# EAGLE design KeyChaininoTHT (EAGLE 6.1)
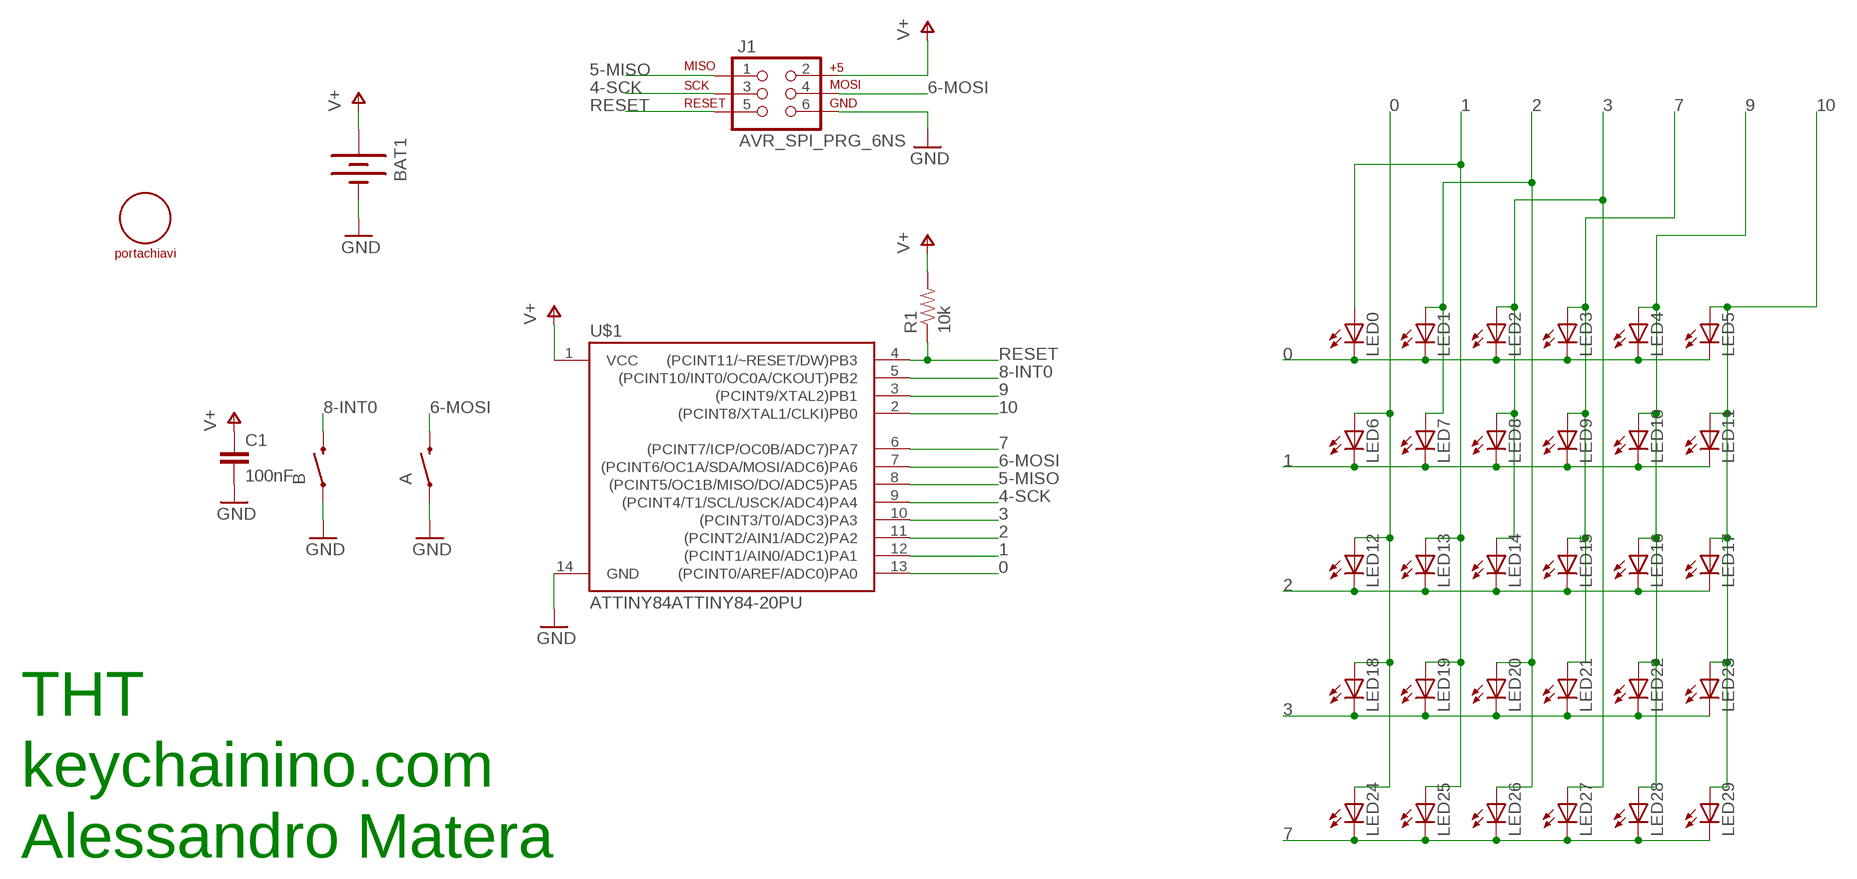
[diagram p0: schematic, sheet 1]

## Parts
A  SWITCH-MOMENTARY-2PTH  [TACTILE-PTH]
B  SWITCH-MOMENTARY-2PTH  [TACTILE-PTH]
BAT1  BATTERY20PTH  [BATTCOM_20MM_PTH]
C1  100nF  CAPPTH1  [CAP-PTH-5MM]
J1  AVR_SPI_PRG_6NS  [2X3-NS]
LED0  LED5MM-KIT  [LED5MM-KIT]
LED1  LED5MM-KIT  [LED5MM-KIT]
LED2  LED5MM-KIT  [LED5MM-KIT]
LED3  LED5MM-KIT  [LED5MM-KIT]
LED4  LED5MM-KIT  [LED5MM-KIT]
LED5  LED5MM-KIT  [LED5MM-KIT]
LED6  LED5MM-KIT  [LED5MM-KIT]
LED7  LED5MM-KIT  [LED5MM-KIT]
LED8  LED5MM-KIT  [LED5MM-KIT]
LED9  LED5MM-KIT  [LED5MM-KIT]
LED10  LED5MM-KIT  [LED5MM-KIT]
LED11  LED5MM-KIT  [LED5MM-KIT]
LED12  LED5MM-KIT  [LED5MM-KIT]
LED13  LED5MM-KIT  [LED5MM-KIT]
LED14  LED5MM-KIT  [LED5MM-KIT]
LED15  LED5MM-KIT  [LED5MM-KIT]
LED16  LED5MM-KIT  [LED5MM-KIT]
LED17  LED5MM-KIT  [LED5MM-KIT]
LED18  LED5MM-KIT  [LED5MM-KIT]
LED19  LED5MM-KIT  [LED5MM-KIT]
LED20  LED5MM-KIT  [LED5MM-KIT]
LED21  LED5MM-KIT  [LED5MM-KIT]
LED22  LED5MM-KIT  [LED5MM-KIT]
LED23  LED5MM-KIT  [LED5MM-KIT]
LED24  LED5MM-KIT  [LED5MM-KIT]
LED25  LED5MM-KIT  [LED5MM-KIT]
LED26  LED5MM-KIT  [LED5MM-KIT]
LED27  LED5MM-KIT  [LED5MM-KIT]
LED28  LED5MM-KIT  [LED5MM-KIT]
LED29  LED5MM-KIT  [LED5MM-KIT]
R1  10k  RESISTORPTH-1/4W  [AXIAL-0.4]
U$1  ATTINY84ATTINY84-20PU  [DIL14]
U$2  ANELLO-PORTACHIAVI  [HOLE-PORTACHIAVI]

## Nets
0: LED0.K(C) LED1.K(C) LED2.K(C) LED3.K(C) LED4.K(C) LED5.K(C) LED6.A LED12.A LED18.A LED24.A U$1.13((PCINT0/AREF/ADC0)PA0)
1: LED0.A LED6.K(C) LED7.K(C) LED8.K(C) LED9.K(C) LED10.K(C) LED11.K(C) LED13.A LED19.A LED25.A U$1.12((PCINT1/AIN0/ADC1)PA1)
2: LED1.A LED7.A LED12.K(C) LED13.K(C) LED14.K(C) LED15.K(C) LED16.K(C) LED17.K(C) LED20.A LED26.A U$1.11((PCINT2/AIN1/ADC2)PA2)
3: LED2.A LED8.A LED14.A LED18.K(C) LED19.K(C) LED20.K(C) LED21.K(C) LED22.K(C) LED23.K(C) LED27.A U$1.10((PCINT3/T0/ADC3)PA3)
4-SCK: J1.3 U$1.9((PCINT4/T1/SCL/USCK/ADC4)PA4)
5-MISO: J1.1 U$1.8((PCINT5/OC1B/MISO/DO/ADC5)PA5)
6-MOSI: A.3 J1.4 U$1.7((PCINT6/OC1A/SDA/MOSI/ADC6)PA6)
7: LED3.A LED9.A LED15.A LED21.A LED24.K(C) LED25.K(C) LED26.K(C) LED27.K(C) LED28.K(C) LED29.K(C) U$1.6((PCINT7/ICP/OC0B/ADC7)PA7)
8-INT0: B.3 U$1.5((PCINT10/INT0/OC0A/CKOUT)PB2)
9: LED4.A LED10.A LED16.A LED22.A LED28.A U$1.3((PCINT9/XTAL2)PB1)
10: LED5.A LED11.A LED17.A LED23.A LED29.A U$1.2((PCINT8/XTAL1/CLKI)PB0)
GND: A.1 B.1 BAT1.2(-) C1.2 J1.6 U$1.14(GND)
RESET: J1.5 R1.P$1 U$1.4((PCINT11/~RESET/DW)PB3)
V+: BAT1.1(+) C1.1 J1.2 R1.P$2 U$1.1(VCC)

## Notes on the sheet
- THT
- keychainino.com
- Alessandro Matera

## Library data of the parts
A B = SparkFun-Electromechanical:SWITCH-MOMENTARY-2: Various NO switches- pushbuttons, reed, etc
BAT1 = SparkFun-Electromechanical:BATTERY: Battery Holders
C1 = SparkFun-Passives:CAP: Capacitor
J1 = SparkFun-Connectors:AVR_SPI_PRG_6: AVR ISP 6 Pin This is the reduced ISP connector for AVR programming. Common on Arduino. This footprint will take up less PCB space and can be used with a 10-pin to 6-pin adapter such as SKU: BOB-08508
LED0 LED1-LED29 = SparkFun-LED:LED: LEDs
R1 = SparkFun-Resistors:RESISTOR: Resistor
U$1 = SparkFun-DigitalIC:ATTINY84: Atmel 14-pin 2/4/8kB flash uC
U$2 = anello-portachiavi:ANELLO-PORTACHIAVI

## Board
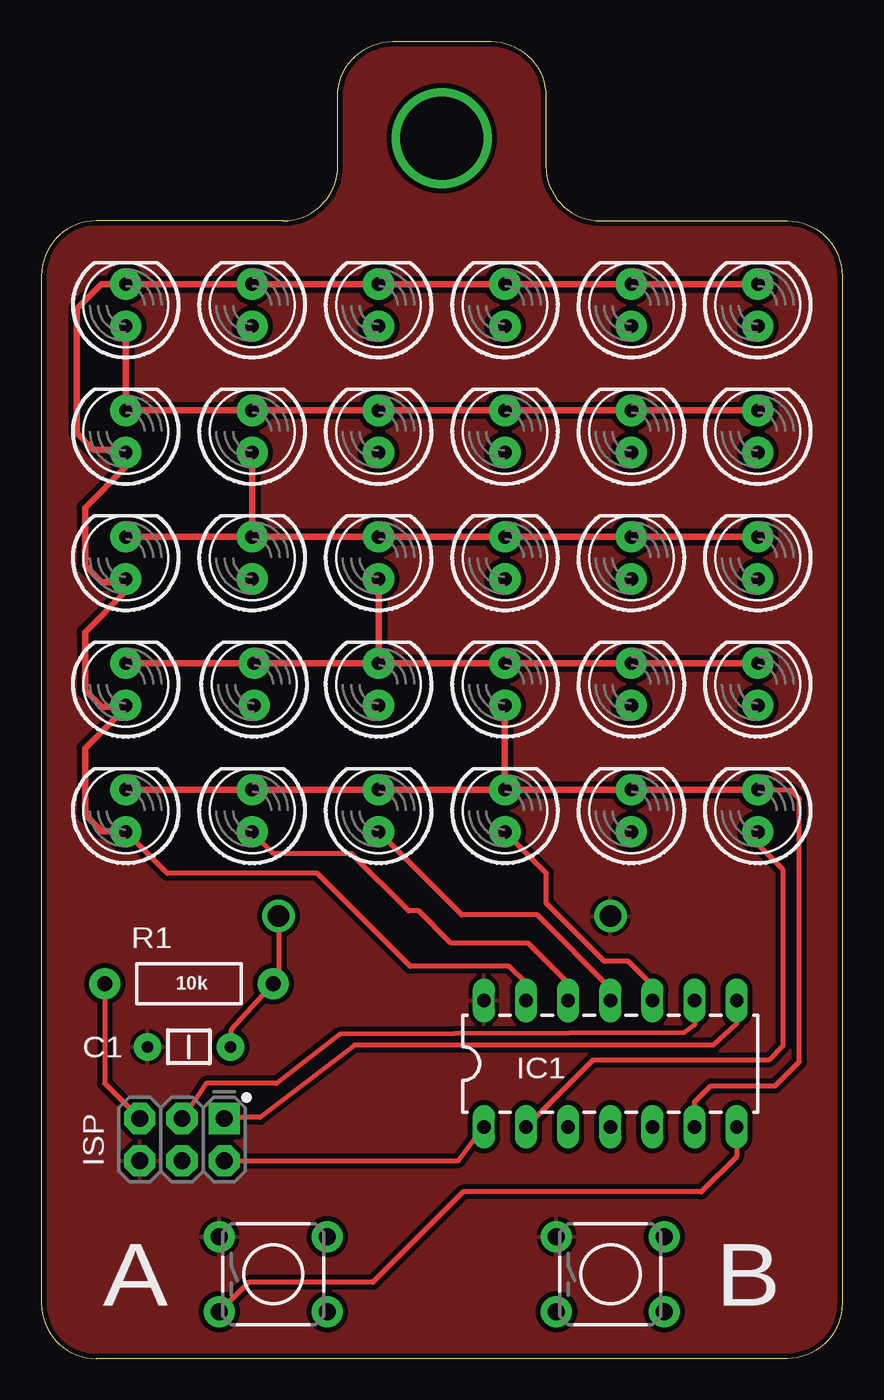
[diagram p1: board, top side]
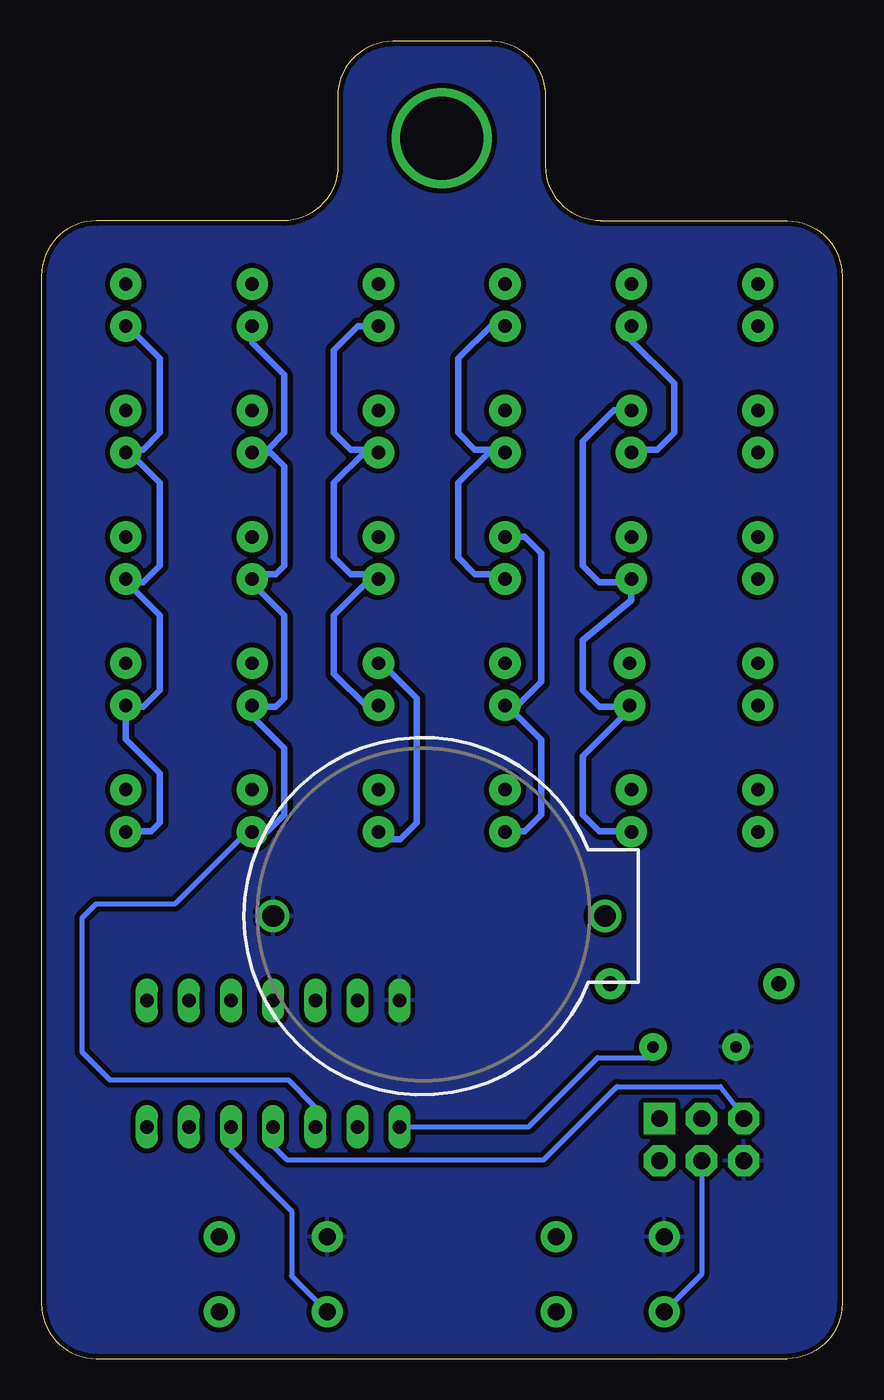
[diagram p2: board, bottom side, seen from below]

Size 48.26 x 79.39 mm. Coordinates in mm from the lower left corner, seen from the top.
Outline: 0,65.28 0,3.3 arc90 3.3,0 44.96,0 arc90 48.26,3.3 48.26,65.28 arc90 44.96,68.58 33.7,68.58 arc-90 30.4,71.88 30.4,76.09 arc90 27.1,79.39 21.16,79.39 arc90 17.86,76.09 17.86,71.88 arc-90 14.56,68.58 3.3,68.58 arc90 0,65.28
Copper layers (1*16): Top 0.035mm / dielectric 1.5mm / Bottom 0.035mm
Design rules: minimum track width 6mil, minimum drill 12mil, track to track 6mil, track to pad 6mil, pad to pad 6mil, via to via 6mil, smd to smd 0mil, copper to edge 10mil, drill to drill 10mil, minimum pad ring 10mil, minimum via ring 6mil, stop-mask expansion 2mil, vias tented up to drill 100mil, thermal gap 10mil

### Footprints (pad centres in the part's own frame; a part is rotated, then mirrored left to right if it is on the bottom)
TACTILE-PTH = drill 1.016 pad 1.88: 1 -3.251,2.261; 2 3.251,2.261; 3 -3.251,-2.261; 4 3.251,-2.261
BATTCOM_20MM_PTH = drill 1.3: 1 20,0; 2 0,0
CAP-PTH-5MM = drill 0.7 pad 1.651: 1 -2.5,0; 2 2.5,0
2X3-NS = drill 1.016 pad 1.88 square: 1 -2.54,-1.27 | drill 1.016 pad 1.88 octagon: 2 -2.54,1.27; 3 0,-1.27; 4 0,1.27; 5 2.54,-1.27; 6 2.54,1.27
LED5MM-KIT = drill 0.813 pad 1.88: A -1.27,0; K 1.27,0
AXIAL-0.4 = drill 0.9 pad 1.88: P$1 -5.08,0; P$2 5.08,0
DIL14 = drill 0.813 long: 1 -8.89,-3.81; 2 -6.35,-3.81; 3 -3.81,-3.81; 4 -1.27,-3.81; 5 1.27,-3.81; 6 3.81,-3.81; 7 6.35,-3.81; 8 6.35,3.81; 9 3.81,3.81; 10 1.27,3.81; 11 -1.27,3.81; 12 -3.81,3.81; 13 -6.35,3.81; 14 -8.89,3.81
HOLE-PORTACHIAVI = drill 5 pad 6: P$1 0,0

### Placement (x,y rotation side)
A  13.97,5.08 0 top
B  34.29,5.08 0 top
BAT1  34.29,26.67 0 bottom
C1  8.89,18.78 180 top
J1  8.47,13.2 180 top
LED0  5.08,63.5 90 top
LED1  12.7,63.5 90 top
LED2  20.32,63.5 90 top
LED3  27.94,63.5 90 top
LED4  35.56,63.5 90 top
LED5  43.18,63.5 90 top
LED6  5.08,55.88 90 top
LED7  12.7,55.88 90 top
LED8  20.32,55.88 90 top
LED9  27.94,55.88 90 top
LED10  35.56,55.88 90 top
LED11  43.18,55.88 90 top
LED12  5.08,48.26 90 top
LED13  12.7,48.26 90 top
LED14  20.32,48.26 90 top
LED15  27.94,48.26 90 top
LED16  35.56,48.26 90 top
LED17  43.18,48.26 90 top
LED18  5.08,40.64 90 top
LED19  12.82,40.64 90 top
LED20  20.32,40.64 90 top
LED21  27.94,40.64 90 top
LED22  35.56,40.64 90 top
LED23  43.18,40.64 90 top
LED24  5.08,33.02 90 top
LED25  12.7,33.02 90 top
LED26  20.32,33.02 90 top
LED27  27.94,33.02 90 top
LED28  35.56,33.02 90 top
LED29  43.18,33.02 90 top
R1  8.89,22.59 0 top
U$1  35.56,17.78 0 top
U$2  24.13,73.56 0 top

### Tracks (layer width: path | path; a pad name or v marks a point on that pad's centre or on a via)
0
  Top 0.305: U$1.13 29.21,22.61 28.18,23.64 22.23,23.64 16.63,29.24 7.59,29.24 LED24.A
  Top 0.406: LED5.K LED4.K LED3.K LED2.K LED1.K LED0.K 3.61,64.77 2.13,63.29 2.13,55.79 3.13,54.79 4.9,54.79 LED6.A | LED24.A 5.04,31.79 3.63,31.79 2.63,32.79 2.63,36.79 5.08,39.24 LED18.A 5,39.29 3.63,39.29 2.63,40.29 2.63,43.79 5.08,46.24 LED12.A 4.88,46.79 3.63,46.79 2.63,47.79 2.63,51.29 5.08,53.74 LED6.A | LED6.A 5.08,54.74 5.13,54.79
1
  Top 0.305: U$1.12 31.75,22.62 29.33,25.04 24.68,25.04 22.73,26.99 22.13,26.99 18.68,30.44 14.01,30.44 LED25.A
  Top 0.406: LED11.K LED10.K LED9.K LED8.K LED7.K LED6.K LED0.A
  Bottom 0.406: LED7.K 13.77,57.15 15.63,55.29 15.63,47.79 14.63,46.79 12.9,46.79 LED13.A 12.7,45.72 15.63,43.29 15.63,40.29 14.63,39.29 12.9,39.29 LED19.A 12.82,39.1 15.63,36.29 15.63,32.79 14.63,31.79 12.74,31.79 LED25.A
2
  Top 0.305: U$1.11 34.29,22.33 29.88,26.74 25.33,26.74 LED26.A
  Top 0.406: LED12.K LED13.K | LED13.K LED14.K LED15.K LED16.K LED17.K | LED7.A LED13.K
  Bottom 0.406: LED1.A 12.7,61.36 10.13,58.79 10.13,55.79 11.13,54.79 12.52,54.79 LED7.A | LED14.K 19.13,49.53 18.13,48.53 18.13,40.79 19.55,39.37 LED20.A 20.21,39.37 18.13,37.29 18.13,32.79 19.13,31.79 20.28,31.79 LED26.A
3
  Top 0.305: U$1.10 36.83,22.49 35.38,23.94 33.93,23.94 30.43,27.44 30.43,29.26 LED27.A
  Top 0.406: LED18.K LED19.K LED20.K | LED20.K LED21.K LED22.K LED23.K | LED14.A LED20.K
  Bottom 0.406: LED2.A 21.19,62.23 23.13,60.29 23.13,55.79 22.13,54.79 20.5,54.79 LED8.A 21.31,54.61 23.13,52.79 23.13,48.29 22.13,47.29 20.62,47.29 LED14.A | LED21.K 27.75,41.91 25.63,39.79 25.63,32.29 26.63,31.29 27.48,31.29 LED27.A
4-SCK
  Top 0.305: U$1.9 39.37,20.13 38.73,19.64 17.98,19.54 14.18,16.59 9.93,16.59 8.53,14.49 8.53,14.09 8.49,13.64 J1.3
5-MISO
  Top 0.305: U$1.8 41.91,20.17 40.48,18.89 18.88,18.89 13.18,14.54 12.08,14.54 J1.1
6-MOSI
  Top 0.305: U$1.7 41.91,12.17 39.78,10.04 25.43,10.04 19.98,4.59 12.49,4.59 A.3
  Bottom 0.305: J1.4 8.47,5.07 A.3
7
  Top 0.305: U$1.6 39.37,15.48 40.33,16.44 44.23,16.44 45.68,17.89 45.68,33.74 45.18,34.24 43.23,34.24 LED29.K
  Top 0.406: LED24.K LED25.K LED26.K LED27.K | LED27.K LED28.K LED29.K | LED21.A LED27.K
  Bottom 0.406: LED3.A 29.19,62.23 30.63,60.79 30.63,55.79 29.63,54.79 28.12,54.79 LED9.A 28.81,54.61 30.63,52.79 30.63,48.29 29.63,47.29 28.24,47.29 LED15.A 28.43,46.99 30.63,44.79 30.63,41.29 28.63,39.29 28.02,39.29 LED21.A
8-INT0
  Bottom 0.305: U$1.5 36.83,12.54 33.18,8.89 33.18,4.96 B.3
9
  Bottom 0.305: LED28.A 35.87,31.75 40.23,27.39 44.98,27.39 45.83,26.54 45.83,18.49 44.13,16.79 33.38,16.79 31.78,15.19 31.78,14 U$1.3
  Bottom 0.406: LED4.A 35.56,61.22 33.63,59.29 33.63,55.79 34.63,54.79 35.38,54.79 LED10.A 34.45,54.61 33.63,53.79 33.63,47.79 34.13,47.29 35.26,47.29 LED16.A 35.56,46.72 33.63,44.79 33.63,39.79 34.13,39.29 35.48,39.29 LED22.A 35.56,38.72 33.63,36.79 33.63,32.79 34.63,31.79 35.52,31.79 LED28.A
10
  Top 0.305: LED29.A 43.18,30.99 44.68,29.49 44.68,18.84 43.83,17.99 33.23,17.99 U$1.2
  Bottom 0.406: LED5.A 43.07,62.23 41.13,60.29 41.13,55.79 42.13,54.79 43,54.79 LED11.A 42.95,54.61 41.13,52.79 41.13,47.79 42.13,46.79 42.98,46.79 LED17.A 43.18,46.84 41.13,44.79 41.13,40.29 42.13,39.29 43.1,39.29 LED23.A 43.18,37.34 41.13,35.29 41.13,32.29 41.63,31.79 43.14,31.79 LED29.A
GND
  pour Top (isolate 0.305): 53.02,-5.16 52.15,83.17 -10.9,84.44 -11.3,-4.59
  pour Bottom (isolate 0.305): 58.64,-3.16 57.27,83.94 -3.24,82.67 -4.41,-5.13
RESET
  Top 0.305: R1.P$1 3.81,16.59 J1.5
  Bottom 0.305: U$1.4 34.29,12.8 33.48,11.99 17.98,11.99 13.58,16.39 7.33,16.39 5.73,14.29 5.73,14.27 J1.5
V+
  Top 0.305: BAT1.1 14.29,21.91 R1.P$2 11.44,19.81 C1.1 | J1.2 25.13,11.93 U$1.1
  Bottom 0.305: U$1.1 18.9,13.97 14.73,18.14 11.75,18.14 C1.1

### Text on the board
tPlace: R1 | C1 | IC1 | ISP | A | B

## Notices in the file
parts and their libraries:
SparkFun-Electromechanical: Licensing: CC v3.0 Share-Alike You are welcome to use this library for commercial purposes.
